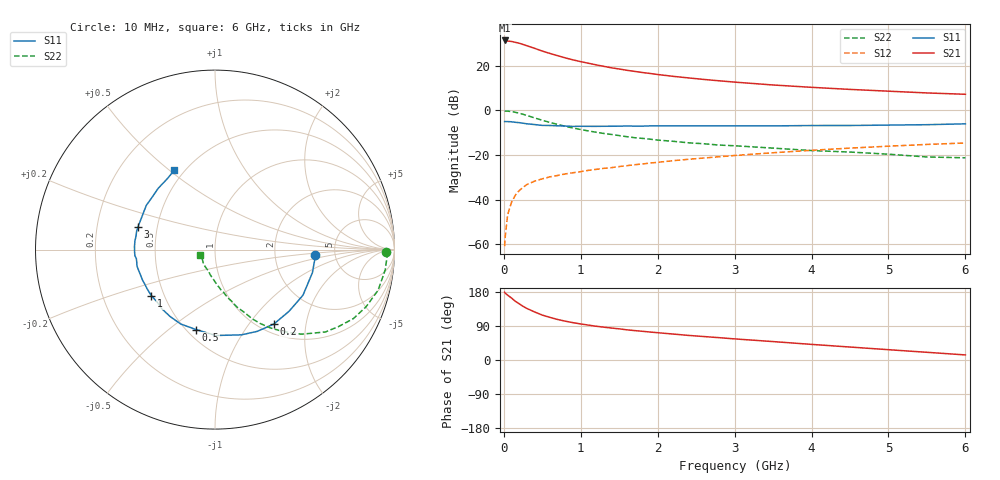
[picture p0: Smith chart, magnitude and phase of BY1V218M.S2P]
! SIEMENS Small Signal Semiconductors
! BFY420
! Si NPN RF SIEGET Grounded Emitter Transistor in MICRO-X
! VCE = 1.25 V  IC = 18 mA
! Common Emitter S-Parameters:  October  1996
# GHz  S  MA  R  50
!  f  S11  S21  S12  S22
! GHz  MAG  ANG  MAG  ANG  MAG  ANG  MAG  ANG
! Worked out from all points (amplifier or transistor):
!   36 points, 10 MHz to 6 GHz, reference 50 ohm
!   highest |S21| = 31.3 dB at 10 MHz (marker M1)
!   |S21| within 3 dB of that: start of sweep to 354.7 MHz
!   unconditionally stable (mu >= 1): 1.943 GHz to end of sweep
!   at 250 MHz: K = 0.28, MSG = 32.0 dB, |S12| = -34.6 dB
!   at 1.4 GHz: K = 0.91, MSG = 22.4 dB, |S12| = -25.7 dB
!   at 6 GHz: K = 1.09, MAG = 9.1 dB, |S12| = -14.7 dB
!   S11 on the Smith chart (normalised r, x): 10 MHz: 3.51, -0.32; 200 MHz: 1.15, -1.33; 500 MHz: 0.56, -0.63; 1 GHz: 0.43, -0.27; 3 GHz: 0.39, +0.12; 6 GHz: 0.44, +0.52
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0.01  0.5601 -3.2  36.73 178.8  0.0009 108.9  0.9538 -0.9
0.02  0.5587 -5.6  36.55 175.9  0.0016 83.8  0.9594 -2.4
0.05  0.5578 -13.3  35.65 171.0  0.0046 82.9  0.9551 -6.8
0.1  0.5522 -27.4  34.87 163.5  0.0087 80.2  0.9364 -14.0
0.15  0.5371 -39.7  33.34 154.8  0.0125 75.1  0.9001 -20.7
0.2  0.5287 -51.7  31.82 148.4  0.0159 70.4  0.8615 -26.5
0.25  0.5127 -62.7  29.84 141.6  0.0187 66.1  0.8112 -31.9
0.3  0.4972 -72.8  27.98 136.0  0.0217 64.4  0.7676 -36.7
0.4  0.4786 -89.5  24.48 126.8  0.0258 59.6  0.6748 -44.3
0.5  0.4579 -103.3  21.23 118.5  0.0291 57.2  0.5967 -50.1
0.6  0.4563 -114.8  18.78 112.4  0.0322 55.0  0.5335 -54.8
0.7  0.4489 -123.9  16.72 106.9  0.0346 54.2  0.4818 -58.6
0.8  0.4431 -131.9  14.93 102.4  0.0375 53.1  0.4364 -61.8
1  0.438 -144.0  12.31 95.1  0.0421 53.5  0.3707 -66.3
1.1  0.4366 -150.0  11.32 92.0  0.0451 53.4  0.3445 -68.9
1.6  0.4443 -168.2  7.878 79.6  0.0573 53.4  0.2558 -77.3
2.2  0.4489 177.7  5.765 68.5  0.0741 52.0  0.2019 -85.7
3  0.4475 163.3  4.279 55.7  0.0971 48.3  0.1603 -94.8
3.5  0.4469 154.9  3.689 48.6  0.1118 45.0  0.1418 -101.1
4.5  0.4561 140.0  2.937 34.2  0.1419 36.7  0.1158 -114.1
5.5  0.4754 124.2  2.447 20.3  0.1716 27.3  0.0898 -141.1
6  0.497 117.1  2.284 13.4  0.1851 22.3  0.0861 -160.3
